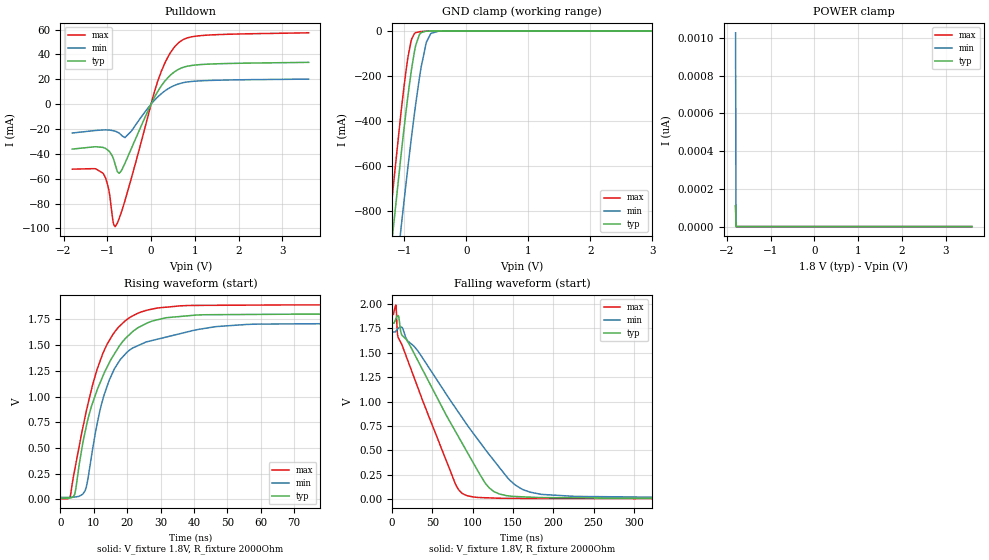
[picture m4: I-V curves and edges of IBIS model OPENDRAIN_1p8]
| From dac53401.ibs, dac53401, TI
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|   OPENDRAIN_1p8 Model
[Model]   OPENDRAIN_1p8
Model_type   I/O_open_drain
Polarity   Non-Inverting
Enable   Active-Low
Vinl = 0.4
Vinh = 1.62
Vmeas = 0.9
Vref = 1.8
Cref = 2pF
Rref = 2000
|   typ   min   max
C_comp   1.258pF   1.229pF   1.287pF
[Voltage Range]   1.8   1.71   1.89
[Temperature Range]   25   125   -40
[Pullup Reference]   1.8   1.71   1.89
[Pulldown Reference]   -0   -0   0
[Power Clamp Reference]   1.8   1.71   1.89
[GND Clamp Reference]   0   0   0
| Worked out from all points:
|   slope of the pulldown table from 0 to 0.27 V, typ, clamps not added: 16.4 ohm
|   GND clamp passes 1 mA (typ) near -0.65 V on its own axis
|   falling waveform, V_fixture 1.8V, R_fixture 2000Ohm: 20-80 % time 70.5ns typ, 86.4ns min, 52.5ns max; typ from 1.8 V to 0.012 V
|   rising waveform, V_fixture 1.8V, R_fixture 2000Ohm: 20-80 % time 10.9ns typ, 9.29ns min, 9.24ns max; typ from 0.012 V to 1.8 V
[Pulldown]
|   Voltage   I(typ)   I(min)   I(max)
-1.8V     -36.15mA   -23.22mA   -52.32mA
-1.098V   -34.82mA   -20.75mA   -55.58mA
-979.2mV  -37.21mA   -20.78mA   -66.6mA
-865.8mV  -43.37mA   -21.34mA   -94.86mA
-817.2mV  -48.87mA   -21.79mA   -98.5mA
-682.2mV  -53.81mA   -24.75mA   -87.4mA
-444.6mV  -35.27mA   -21.46mA   -58.93mA
160.2mV   10.68mA    6.088mA    19.27mA
387mV     21.43mA    12.35mA    38.11mA
613.8mV   27.79mA    16.14mA    48.97mA
1.143V    31.91mA    18.82mA    55.22mA
3.6V      33.67mA    20.17mA    57.45mA
[GND Clamp]
|   Voltage   I(typ)   I(min)   I(max)
-1.8V     -2.596A    -2.851A    -2.471A
-1.433V   -1.564A    -1.858A    -1.402A
-1.201V   -928.8mA   -1.245A    -744.2mA
-1.179V   -871.1mA   -1.189A    -684.9mA
-1.055V   -548.9mA   -872.2mA   -358.3mA
-941.4mV  -281.8mA   -596mA     -112.3mA
-882mV    -162.3mA   -459.7mA   -34.2mA
-822.6mV  -68.79mA   -332mA     -7.838mA
-757.8mV  -15.19mA   -206.4mA   -2.984mA
-644.4mV  -611.1uA   -48.59mA   -607.3uA
-444.6mV  -4.804uA   -314.9uA   -3.221uA
3.6V      0A         0A         0A
[POWER Clamp]
|   Voltage   I(typ)   I(min)   I(max)
-1.8V     109.3pA    1.028nA    111pA
-1.789V   0A         0A         0A
-1.784V   0A         0A         0A
3.6V      0A         0A         0A
[Ramp]
R_load = 2000
|   typ   min   max
dV/dt_r   1.07282/1.08624e-08   1.01393/9.23116e-09   1.12988/9.2542e-09
dV/dt_f   1.07282/7.03748e-08   1.01391/8.57477e-08   1.12988/5.24625e-08
[Falling Waveform]
V_fixture = 1.8V
V_fixture_min = 1.71V
V_fixture_max = 1.89V
R_fixture = 2000Ohm
C_fixture = 0F
|   Time   V(typ)   V(min)   V(max)
0s        1.8V       1.71V      1.89V
4.646ns   1.845V     1.719V     1.988V
7.422ns   1.879V     1.748V     1.657V
12.07ns   1.68V      1.76V      1.583V
78.53ns   695.1mV    936.2mV    158mV
100.3ns   378.8mV    679.9mV    24.79mV
120.3ns   118.6mV    459.6mV    15.15mV
152.8ns   29.52mV    146.2mV    10.18mV
226.9ns   15.67mV    30.27mV    7.485mV
1.5us     11.97mV    20.15mV    6.861mV
[Rising Waveform]
V_fixture = 1.8V
V_fixture_min = 1.71V
V_fixture_max = 1.89V
R_fixture = 2000Ohm
C_fixture = 0F
|   Time   V(typ)   V(min)   V(max)
0s        11.96mV    20.12mV    6.859mV
2.913ns   14.36mV    20.15mV    27.5mV
4.236ns   47.13mV    22.99mV    281.4mV
7.365ns   652.5mV    83.69mV    800.3mV
11.76ns   1.124V     853.2mV    1.334V
15.61ns   1.385V     1.23V      1.598V
23.2ns    1.668V     1.494V     1.809V
36.28ns   1.779V     1.614V     1.882V
90.43ns   1.8V       1.71V      1.89V
1.5us     1.8V       1.71V      1.89V
